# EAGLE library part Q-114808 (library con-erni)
Male Connector SMC-Q 80 contacts Standard Assembly Height Source: http://www.erni.com/DB/PDF-Drawing/SMC/114808.pdf
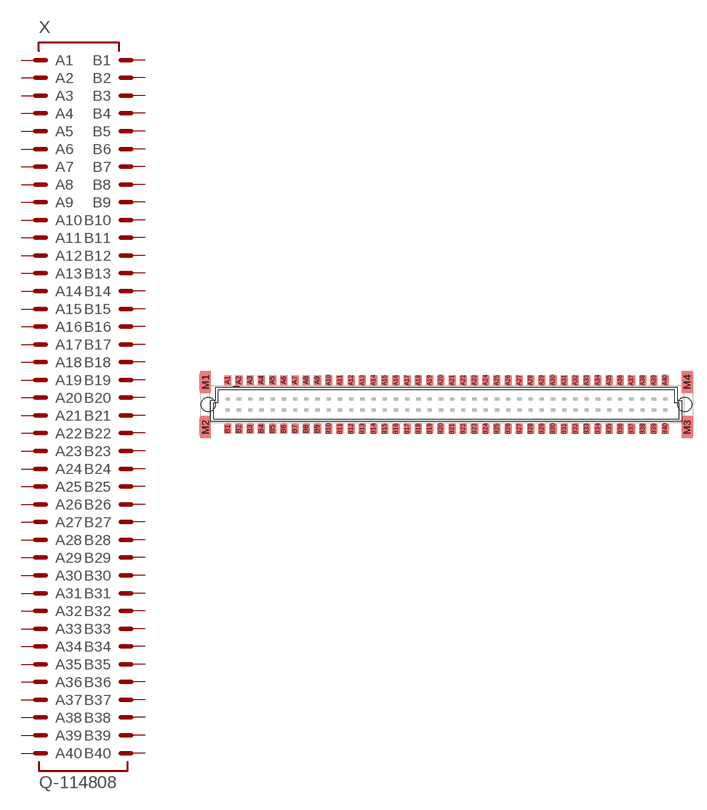
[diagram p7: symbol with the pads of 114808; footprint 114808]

Designator prefix X

## Q-114808 (OC_FARNELL: unknown; OC_NEWARK: unknown)  [114808]
A1  A1  pas
A2  A2  pas
A3  A3  pas
A4  A4  pas
A5  A5  pas
A6  A6  pas
A7  A7  pas
A8  A8  pas
A9  A9  pas
A10  A10  pas
A11  A11  pas
A12  A12  pas
A13  A13  pas
A14  A14  pas
A15  A15  pas
A16  A16  pas
A17  A17  pas
A18  A18  pas
A19  A19  pas
A20  A20  pas
A21  A21  pas
A22  A22  pas
A23  A23  pas
A24  A24  pas
A25  A25  pas
A26  A26  pas
A27  A27  pas
A28  A28  pas
A29  A29  pas
A30  A30  pas
A31  A31  pas
A32  A32  pas
A33  A33  pas
A34  A34  pas
A35  A35  pas
A36  A36  pas
A37  A37  pas
A38  A38  pas
A39  A39  pas
A40  A40  pas
B1  B1  pas
B2  B2  pas
B3  B3  pas
B4  B4  pas
B5  B5  pas
B6  B6  pas
B7  B7  pas
B8  B8  pas
B9  B9  pas
B10  B10  pas
B11  B11  pas
B12  B12  pas
B13  B13  pas
B14  B14  pas
B15  B15  pas
B16  B16  pas
B17  B17  pas
B18  B18  pas
B19  B19  pas
B20  B20  pas
B21  B21  pas
B22  B22  pas
B23  B23  pas
B24  B24  pas
B25  B25  pas
B26  B26  pas
B27  B27  pas
B28  B28  pas
B29  B29  pas
B30  B30  pas
B31  B31  pas
B32  B32  pas
B33  B33  pas
B34  B34  pas
B35  B35  pas
B36  B36  pas
B37  B37  pas
B38  B38  pas
B39  B39  pas
B40  B40  pas

## Footprint 114808 (pad centres in mm)
Male Connector SMC-Q 80 contacts Standard Assembly Height Source: http://www.erni.com/DB/PDF-Drawing/SMC/114808.pdf
smd 0.8 x 1.1: A1 -24.765,2.765; A2 -23.495,2.765; A3 -22.225,2.765; A4 -20.955,2.765; A5 -19.685,2.765; A6 -18.415,2.765; A7 -17.145,2.765; A8 -15.875,2.765; A9 -14.605,2.765; A10 -13.335,2.765; A11 -12.065,2.765; A12 -10.795,2.765; A13 -9.525,2.765; A14 -8.255,2.765; A15 -6.985,2.765; A16 -5.715,2.765; A17 -4.445,2.765; A18 -3.175,2.765; A19 -1.905,2.765; A20 -0.635,2.765; A21 0.635,2.765; A22 1.905,2.765; A23 3.175,2.765; A24 4.445,2.765; A25 5.715,2.765; A26 6.985,2.765; A27 8.255,2.765; A28 9.525,2.765; A29 10.795,2.765; A30 12.065,2.765; A31 13.335,2.765; A32 14.605,2.765; A33 15.875,2.765; A34 17.145,2.765; A35 18.415,2.765; A36 19.685,2.765; A37 20.955,2.765; A38 22.225,2.765; A39 23.495,2.765; A40 24.765,2.765; B1 -24.765,-2.74; B2 -23.495,-2.74; B3 -22.225,-2.74; B4 -20.955,-2.74; B5 -19.685,-2.74; B6 -18.415,-2.74; B7 -17.145,-2.74; B8 -15.875,-2.74; B9 -14.605,-2.74; B10 -13.335,-2.74; B11 -12.065,-2.74; B12 -10.795,-2.74; B13 -9.525,-2.74; B14 -8.255,-2.74; B15 -6.985,-2.74; B16 -5.715,-2.74; B17 -4.445,-2.74; B18 -3.175,-2.74; B19 -1.905,-2.74; B20 -0.635,-2.74; B21 0.635,-2.74; B22 1.905,-2.74; B23 3.175,-2.74; B24 4.445,-2.74; B25 5.715,-2.74; B26 6.985,-2.74; B27 8.255,-2.74; B28 9.525,-2.74; B29 10.795,-2.74; B30 12.065,-2.74; B31 13.335,-2.74; B32 14.605,-2.74; B33 15.875,-2.74; B34 17.145,-2.74; B35 18.415,-2.74; B36 19.685,-2.74; B37 20.955,-2.74; B38 22.225,-2.74; B39 23.495,-2.74; B40 24.765,-2.74
smd 1.2 x 2.5: M1 -27.27,2.55; M2 -27.27,-2.55; M3 27.27,-2.55; M4 27.27,2.55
